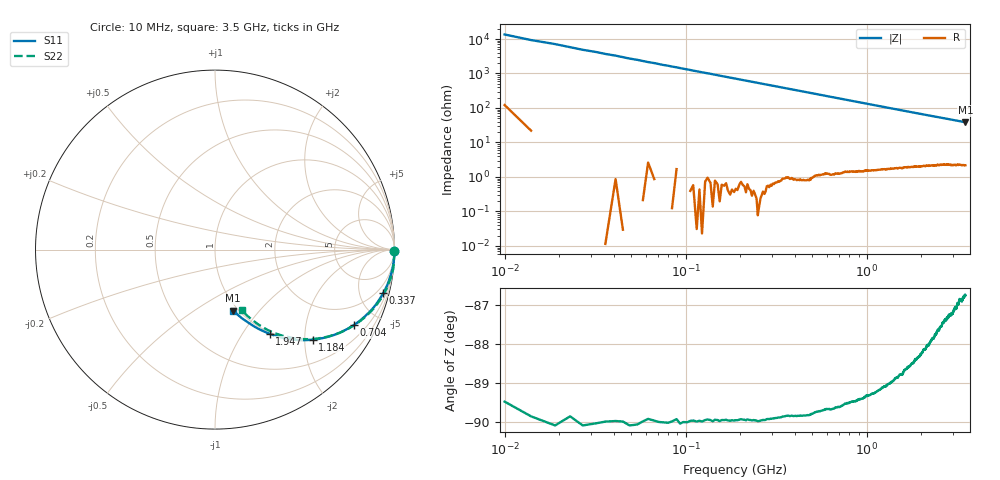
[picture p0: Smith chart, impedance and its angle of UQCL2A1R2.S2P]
! AVX Corporation
! Date:  10/27/06
! Part No:  UQCL2A1R2
! Description:  Ultra Low ESR Microwave capacitors
! Mounting Orientation:  Horizontal
# GHZ S DB R 50
! Freq  |S11|  S11 Ph  |S21|  S21 Ph  |S12|  S12 Ph  |S22|  S22 Ph
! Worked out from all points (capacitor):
!   801 points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, 10 MHz to 3.5 GHz, reference 50 ohm
!   read as one part in series: C = 1.19 pF near 27 MHz
!   lowest |Z| = 38.5 ohm at 3.5 GHz (marker M1)
!   S11 on the Smith chart (normalised r, x): 10 MHz: open; 337 MHz: 0.98, -7.69; 704 MHz: 0.98, -3.68; 1.184 GHz: 0.98, -2.18; 1.947 GHz: 0.98, -1.33; 3.5 GHz: 0.94, -0.73
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0.01  -0.01 -0.5  -42.64 89.0  -42.36 89.9  -0.01 -0.6
0.019  -0.01 -0.9  -37.06 89.2  -37.04 88.9  -0.01 -0.8
0.036  0.00 -1.7  -31.35 88.4  -31.33 88.5  -0.01 -1.6
0.049  -0.01 -2.2  -28.66 87.9  -28.65 87.8  -0.01 -2.1
0.075  -0.02 -3.4  -24.98 86.7  -24.93 86.7  -0.01 -3.3
0.11  -0.03 -4.9  -21.69 85.1  -21.65 85.1  -0.01 -4.8
0.158  -0.07 -7.0  -18.58 83.0  -18.54 83.0  -0.03 -6.9
0.206  -0.11 -9.1  -16.32 80.9  -16.28 80.9  -0.07 -8.9
0.267  -0.18 -11.7  -14.14 78.3  -14.10 78.3  -0.13 -11.5
0.337  -0.28 -14.6  -12.22 75.4  -12.18 75.3  -0.23 -14.4
0.459  -0.51 -19.6  -9.76 70.4  -9.72 70.3  -0.46 -19.3
0.595  -0.83 -24.7  -7.82 65.1  -7.79 65.0  -0.77 -24.4
0.704  -1.11 -28.6  -6.66 61.2  -6.62 61.1  -1.06 -28.2
0.917  -1.75 -35.5  -5.01 54.2  -4.97 54.2  -1.70 -35.0
1.175  -2.58 -42.5  -3.71 47.2  -3.68 47.1  -2.53 -41.7
1.184  -2.61 -42.7  -3.68 47.0  -3.65 46.9  -2.56 -41.9
1.471  -3.56 -49.0  -2.78 40.6  -2.74 40.5  -3.50 -47.8
1.755  -4.47 -54.1  -2.20 35.6  -2.17 35.5  -4.39 -52.3
1.947  -5.05 -57.1  -1.92 32.8  -1.90 32.7  -4.96 -54.9
2.34  -6.17 -62.2  -1.53 28.1  -1.50 28.1  -6.05 -59.0
2.92  -7.64 -68.2  -1.20 23.2  -1.17 23.1  -7.46 -63.2
3.5  -9.01 -73.7  -1.02 19.6  -0.99 19.5  -8.68 -66.3
